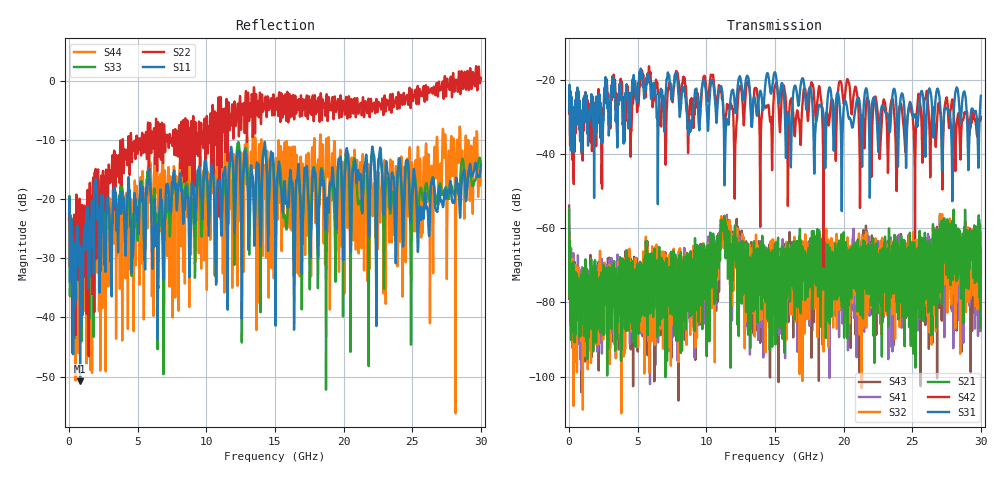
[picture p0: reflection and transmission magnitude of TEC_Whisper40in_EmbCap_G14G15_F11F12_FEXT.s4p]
! Tyco Electronics
! F11F12-G14G15_FEXT
!! PART DESCRIPTION: Whisper 40in Megtron 6 VLP-HVLP-VLP Channel, Embedded Capactior Connecter at one end, bulkhead 2.4mm test pts
!! MODEL DESCRIPTION: System 4-port S-parameter
!! MODEL STATUS: Measured
!! MODEL GEOMETRY: Channel Model
!! MODEL FREQUENCY RANGE: DC to 30.000 GHz in 10.000 MHz frequency steps
!! MODEL EDGE RATE LIMITATION: 12.500 ps (Using conservative 0.5/Fmax rule of thumb)
!! TIME-DOMAIN TRANSFORM CAUTIONS:
!! 1.) Do not simulate transient edge rates faster than the number listed above.  Edge rates faster than this number
!!  contain significant spectral content at frequencies above the model's highest frequency.
!! 2.) Even when simulating edge rates that are slower than the number listed above, be aware that the best time
!!  resolution possible with a direct iFFT is (1 / 2Fmax).  As a result, time resolution is typically not adequate
!!  for most time-domain simulations unless tricks such as windowing are used to minimize leakage and aliasing.
!! 3.) Because the model has a uniform frequency step, a direct iFFT will result in an impulse that that has a time
!!  length given by either (1 / Fstep) or (1 / 2Fstep), depending on the transform being used.  Care has been taken
!!  in selecting the frequency step to ensure a settled impulse response for the model.  Therefore, convolution with
!!  the model's impulse response should present no issues.  However, if directly concatenating s-parameter models
!!  in the frequency domain a user must either interpolate necessary interim frequencies or complete impulse response
!!  zero-padding.  Impulse response zero-padding is more difficult, but more accurate.
!! PORT DEFINITIONS:
!! Port  1  ----->  Side A  F11  G14  Side B  <-----  Port  2
!! Port  3  ----->  Side A  F12  G15  Side B  <-----  Port  4
! Point-to-Point link (differential)  !
! Connectors:  !
!  1: STRADA Whisper  !
! Materials:  !
!  Backplane: Megtron-6 HVLP  !
!  Daughtercard: Megtron-6 VLP  !
! Stack-up:  !
!  Backplane: 20 layers, 200mil thick  !
!  Daughtercard: 14 layers, 110mil thick  !
! Trace Length:  !
!  Backplane: 30in  !
!  Daightercards: 5in  !
! Trace Width:  !
!  Backplane: 7-9-7 mils  !
!  Daughtercards: 6-9-6 mils  !
! Geometry:  !
!  Backplane: Stripline  !
!  Daughtercards: Stripline  !
! Freq. Range: 0 GHz - 30 GHz  !
! Note1: non-mixed-mode s-parameters  !
! Note2: channel includes 2.4mm test points  !
! Touchstone data
! Created: 02-Jul-2013 by IdEM R2011 (7.0.3)
# Hz S MA R 50
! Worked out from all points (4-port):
!   3000 points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, 10 MHz to 30 GHz, reference 50 ohm
!   strongest paths, dB at 10 MHz, 7.51 GHz, 15.01 GHz, 22.51 GHz, 30 GHz:
!     S31: -28.2, -24.9, -17.9, -38.2, -24.2
!     S42: -28.9, -24.7, -21.6, -30.4, -29.9
!     S21: -54.9, -70.6, -67.7, -74.5, -68.4
!     S32: -64.0, -75.6, -72.1, -74.8, -62.3
!     S41: -64.8, -78.0, -74.3, -63.4, -63.3
!     S43: -53.8, -82.7, -70.8, -67.7, -66.1
!   lowest |S11| = -50.8 dB at 810 MHz (marker M1), VSWR 1.01, Z = 49.9 + j0.275 ohm
!   |S11| at or under -10 dB: start of sweep to end of sweep
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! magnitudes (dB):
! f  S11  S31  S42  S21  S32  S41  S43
! 10 MHz  -22.5  -28.2  -28.9  -54.9  -64.0  -64.8  -53.8
! 810 MHz  -50.8  -36.4  -35.7  -76.4  -88.7  -72.7  -87.6
! 1.98 GHz  -17.1  -24.4  -37.8  -85.2  -72.6  -91.0  -74.3
! 10.05 GHz  -16.8  -28.6  -24.0  -80.0  -72.8  -71.8  -72.8
! 11.22 GHz  -16.3  -26.5  -26.7  -58.1  -61.9  -60.1  -64.1
! 13.23 GHz  -14.8  -27.6  -26.5  -71.7  -73.5  -66.1  -79.3
! 30 GHz  -14.3  -24.2  -29.9  -68.4  -62.3  -63.3  -66.1
